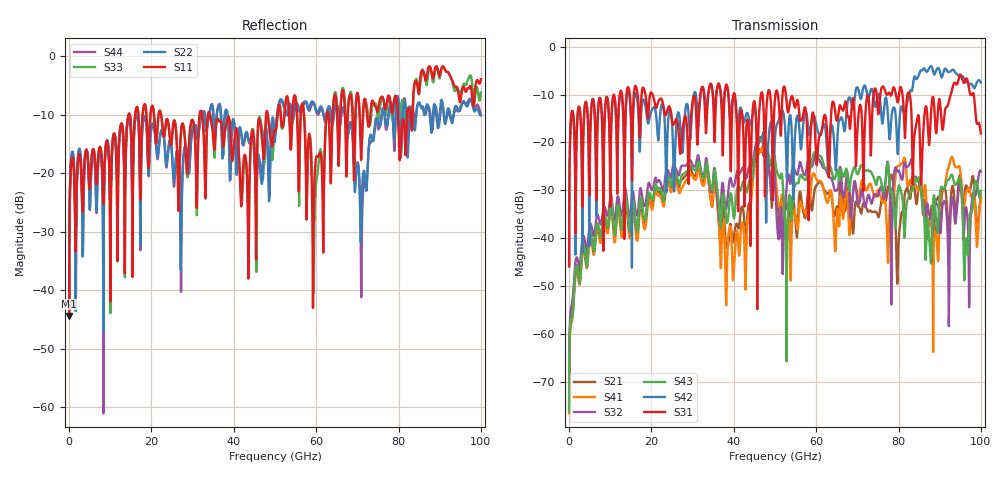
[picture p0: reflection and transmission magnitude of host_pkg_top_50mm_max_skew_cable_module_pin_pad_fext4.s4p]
# Hz S RI R 50
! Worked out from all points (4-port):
!   10000 points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, 10 MHz to 100 GHz, reference 50 ohm
!   strongest paths, dB at 10 MHz, 25.01 GHz, 50.01 GHz, 75.01 GHz, 100 GHz:
!     S31: -45.9, -15.7, -10.8, -13.8, -18.1
!     S42: -45.9, -16.0, -18.9, -10.1, -7.5
!     S43: -76.1, -28.2, -23.6, -27.3, -30.1
!     S32: -75.0, -26.0, -28.7, -31.2, -26.1
!     S41: -76.6, -29.5, -26.3, -29.9, -31.4
!     S21: -75.8, -28.3, -26.5, -35.4, -31.7
!   lowest |S11| = -44.4 dB at 10 MHz (marker M1), VSWR 1.01, Z = 50.3 + j0.535 ohm
!   |S11| at or under -10 dB: start of sweep to 14.44 GHz; 22.33 GHz to 31.7 GHz (9.366 GHz wide, 34.7 % of centre); 34.19 GHz to 47.84 GHz (13.65 GHz wide, 33.3 % of centre)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
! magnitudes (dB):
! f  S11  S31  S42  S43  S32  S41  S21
! 10 MHz  -44.4  -45.9  -45.9  -76.1  -75.0  -76.6  -75.8
! 3.44 GHz  -23.2  -19.3  -18.7  -41.4  -39.6  -42.6  -41.3
! 25.62 GHz  -11.0  -15.9  -26.6  -26.1  -24.8  -27.7  -26.9
! 54.86 GHz  -6.8  -12.7  -18.6  -28.9  -26.0  -34.9  -35.2
! 59.55 GHz  -22.3  -15.5  -14.6  -22.1  -23.2  -26.6  -30.3
! 71.05 GHz  -15.9  -14.2  -10.4  -24.8  -29.9  -28.0  -34.6
! 100 GHz  -3.9  -18.1  -7.5  -30.1  -26.1  -31.4  -31.7
